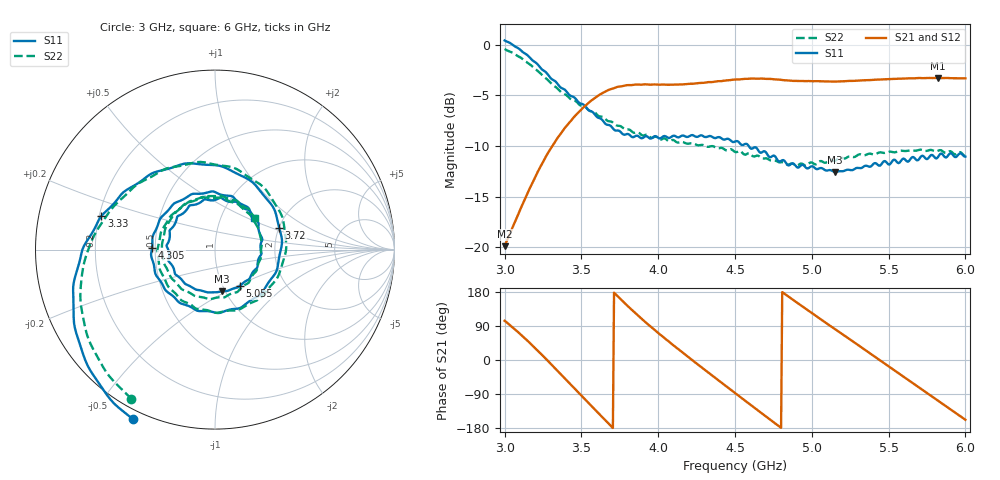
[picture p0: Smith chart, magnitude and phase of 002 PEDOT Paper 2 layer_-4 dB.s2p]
!  04/11/2025  18:37:47
! Ref Plane: 0.000 mm
# MHZ S MA R  50
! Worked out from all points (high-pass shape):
!   401 points, 3 GHz to 6 GHz, reference 50 ohm
!   highest |S21| = -3.27 dB at 5.82 GHz (marker M1); lowest = -19.9 dB at 3 GHz (marker M2)
!   |S21| within 3 dB of the highest: 3.507 GHz to end of sweep
!   lowest |S11| = -12.6 dB at 5.152 GHz (marker M3), VSWR 1.62, Z = 48.3 - j23.8 ohm
!   |S11| at or under -10 dB: 4.59 GHz to end of sweep
!   |S22| runs from -11.9 to -0.4 dB; largest |S21 - S12| = 0.011
!   S11 on the Smith chart (normalised r, x): 3 GHz: -0.03, -0.63; 3.33 GHz: 0.21, +0.14; 3.72 GHz: 2.00, +0.57; 4.305 GHz: 0.48, +0.01; 5.055 GHz: 1.20, -0.52; 6 GHz: 1.43, +0.55
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3000  1.05 -115.8  0.1014 103.5  0.1023 104.3  0.953 -119.3
3150  0.8865 -152.3  0.1856 50.5  0.1858 51.3  0.8147 -155.8
3330  0.6604 163.6  0.3341 -22.4  0.3349 -21.9  0.621 158.9
3502.5  0.511 112.2  0.4818 -95.1  0.4828 -95.0  0.4993 107.1
3600  0.441 74.3  0.5546 -135.9  0.5565 -135.8  0.4531 69.7
3720  0.3777 19.0  0.6142 174.7  0.6156 175.1  0.4035 16.5
3870  0.3542 -46.8  0.6358 116.7  0.6394 117.5  0.3691 -48.1
4005  0.3453 -94.0  0.6352 69.6  0.6361 70.3  0.3431 -94.9
4162.5  0.3566 -141.0  0.6374 18.4  0.641 18.8  0.3309 -143.5
4305  0.3505 178.2  0.6503 -26.6  0.653 -25.7  0.317 176.6
4500  0.3329 116.2  0.6737 -87.0  0.6775 -86.5  0.2958 113.7
4612.5  0.3072 78.8  0.6811 -121.7  0.6833 -121.5  0.283 76.2
4755  0.2836 31.3  0.6751 -165.4  0.6761 -164.8  0.2686 26.5
4867.5  0.2589 -3.3  0.6646 161.7  0.6646 162.3  0.2595 -8.7
5002.5  0.2514 -40.7  0.6607 123.3  0.6608 123.8  0.2619 -46.2
5055  0.2462 -55.9  0.6607 108.4  0.6606 108.8  0.2667 -61.7
5152.5  0.2354 -80.4  0.6579 81.0  0.6583 81.4  0.2673 -87.5
5347.5  0.2529 -130.7  0.6685 26.4  0.6701 26.8  0.2852 -141.0
5505  0.2561 -175.4  0.6765 -17.9  0.6797 -17.2  0.2965 176.7
5677.5  0.2716 134.2  0.6843 -66.7  0.6881 -65.9  0.2999 127.9
5820  0.2782 88.9  0.6865 -107.2  0.6903 -106.5  0.2996 86.9
6000  0.2806 39.5  0.6828 -157.8  0.6855 -157.3  0.2825 38.8
